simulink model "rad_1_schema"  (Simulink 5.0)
settings: Solver=ode45  StartTime=0.0  StopTime=10.0  RelTol=1e-3

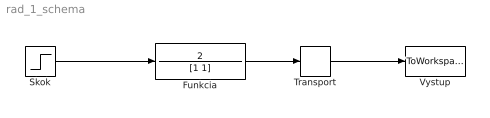
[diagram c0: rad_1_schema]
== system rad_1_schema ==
  Funkcia : TransferFcn  Numerator=2  Denominator=[1 1]
  Skok : Step  Time=0  SampleTime=0
  Transport : TransportDelay  DelayTime=3
  Vystup : ToWorkspace  VariableName=yout  SampleTime=-1  SaveFormat=Array
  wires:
  Funkcia/1 -> Transport/1
  Transport/1 -> Vystup/1
  Skok/1 -> Funkcia/1
